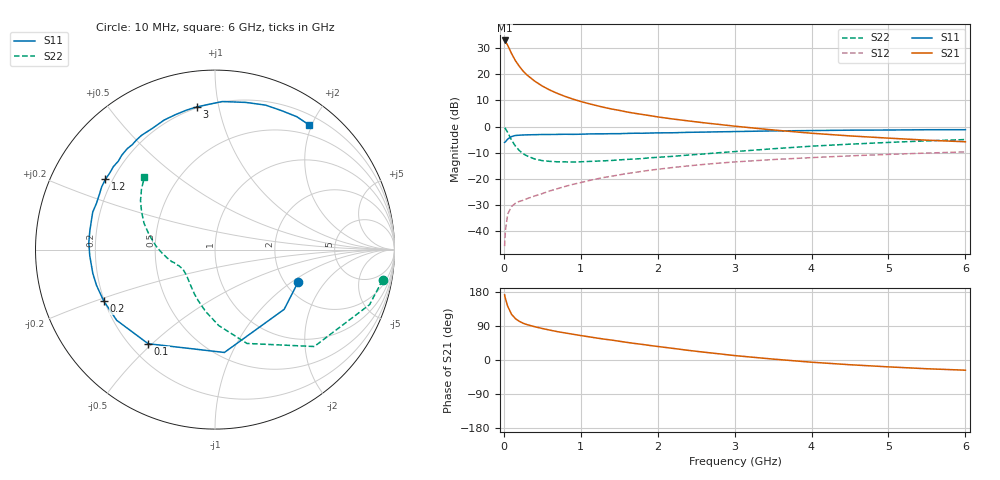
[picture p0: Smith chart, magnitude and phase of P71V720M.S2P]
! SIEMENS Small Signal Semiconductors
! BFP196
! Si NPN RF Bipolar Junction Transistor in SOT143
! VCE = 1.75 V  IC = 20 mA
! Common Emitter S-Parameters:  May  1996
# GHz  S  MA  R  50
!  f  S11  S21  S12  S22
! GHz  MAG  ANG  MAG  ANG  MAG  ANG  MAG  ANG
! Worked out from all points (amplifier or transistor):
!   36 points, 10 MHz to 6 GHz, reference 50 ohm
!   highest |S21| = 33.0 dB at 10 MHz (marker M1)
!   |S21| within 3 dB of that: start of sweep to 68.29 MHz
!   unconditionally stable (mu >= 1): 644.7 MHz to 3.494 GHz; 3.543 GHz to 4.074 GHz
!   at 250 MHz: K = 0.62, MSG = 24.8 dB, |S12| = -28.3 dB
!   at 1.4 GHz: K = 1.12, MAG = 10.8 dB, |S12| = -19.0 dB
!   at 6 GHz: K = 0.98, MSG = 1.9 dB, |S12| = -9.7 dB
!   S11 on the Smith chart (normalised r, x): 10 MHz: 2.34, -1.13; 100 MHz: 0.27, -0.49; 200 MHz: 0.20, -0.21; 1.2 GHz: 0.17, +0.29; 3 GHz: 0.19, +0.86; 6 GHz: 0.34, +1.97
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0.01  0.497 -21.5  44.7 171.8  0.0051 84.0  0.949 -10.3
0.02  0.5092 -40.8  42.88 162.4  0.01 74.9  0.9142 -19.6
0.05  0.5755 -84.8  36.14 141.8  0.021 58.6  0.7731 -44.3
0.1  0.6433 -125.4  25.14 120.7  0.0294 44.1  0.5523 -71.2
0.15  0.6747 -144.3  18.37 109.2  0.0338 40.1  0.4235 -87.2
0.2  0.6829 -155.3  14.36 102.1  0.0367 39.9  0.3488 -98.6
0.25  0.6896 -163.2  11.61 97.1  0.0386 40.4  0.3014 -107.7
0.3  0.6936 -169.0  9.782 93.5  0.0414 42.0  0.2748 -114.3
0.4  0.6986 -177.2  7.447 87.9  0.0467 45.0  0.2394 -124.9
0.5  0.7042 176.9  5.974 83.1  0.0519 47.2  0.2223 -132.4
0.6  0.7052 171.4  4.993 78.8  0.0586 49.7  0.215 -137.7
0.7  0.7077 166.5  4.296 74.7  0.0646 50.9  0.211 -141.7
0.9  0.7089 158.6  3.352 67.9  0.0782 52.5  0.2088 -148.0
1.1  0.7216 151.1  2.758 61.4  0.0918 52.8  0.2145 -152.2
1.2  0.7255 147.3  2.534 58.2  0.0987 52.5  0.2175 -154.2
1.6  0.7394 134.5  1.902 46.5  0.1257 49.7  0.2349 -160.5
2.2  0.7606 117.1  1.394 30.6  0.1642 43.5  0.269 -169.7
3  0.8017 97.2  1.018 11.7  0.2099 33.5  0.3314 176.1
3.5  0.8259 87.2  0.861 2.4  0.2332 27.2  0.3756 167.4
4.5  0.8529 70.7  0.662 -12.5  0.2745 15.8  0.46 152.8
5.5  0.8694 58.4  0.548 -23.1  0.3107 5.0  0.532 140.3
6  0.8705 52.8  0.511 -26.9  0.3271 -0.9  0.5637 134.2
